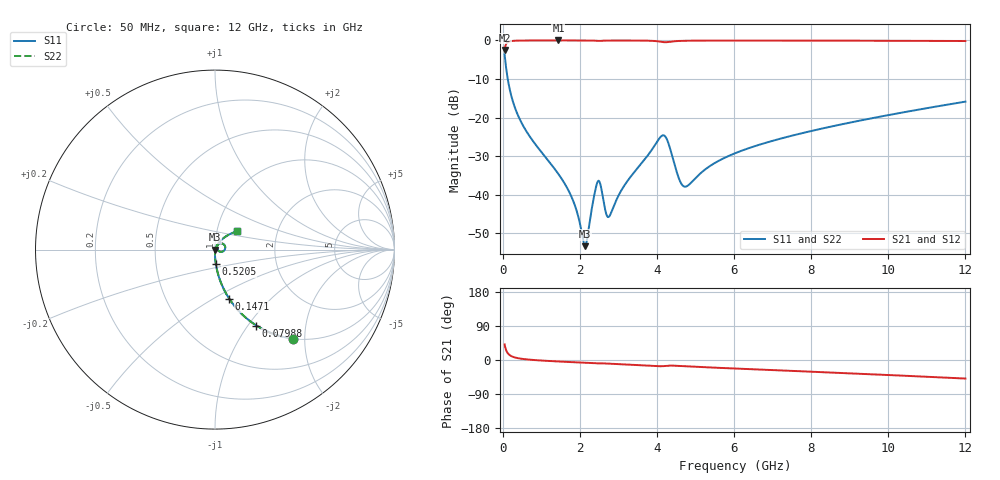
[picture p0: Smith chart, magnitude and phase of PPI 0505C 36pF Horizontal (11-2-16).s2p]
# MHz S MA R 50
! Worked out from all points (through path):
!   1601 points, 50 MHz to 12 GHz, reference 50 ohm
!   highest |S21| = -0.01 dB at 1.447 GHz (marker M1); lowest = -2.5 dB at 50 MHz (marker M2)
!   group delay of S21, straight-line fit = 12.2 ps
!   lowest |S11| = -53.3 dB at 2.134 GHz (marker M3), VSWR 1.00, Z = 50.2 - j0.0716 ohm
!   |S11| at or under -10 dB: 131.4 MHz to end of sweep
!   |S22| runs from -53.3 to -3.6 dB; largest |S21 - S12| = 0
!   S11 on the Smith chart (normalised r, x): 50 MHz: 1.00, -1.75; 79.88 MHz: 1.00, -1.10; 147.1 MHz: 1.00, -0.59; 520.5 MHz: 1.00, -0.16; 12 GHz: 1.25, +0.26
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50  0.6599 -48.9  0.7511 41.1  0.7511 41.1  0.6599 -48.9
79.875  0.4815 -61.5  0.8761 28.5  0.8761 28.5  0.4815 -61.5
147.0938  0.2852 -73.9  0.958 16.1  0.958 16.1  0.2852 -73.9
296.4688  0.1443 -82.5  0.9889 7.3  0.9889 7.3  0.1443 -82.5
520.5312  0.08008 -86.7  0.996 2.8  0.996 2.8  0.08008 -86.7
1446.656  0.01856 -90.1  0.9985 -3.9  0.9985 -3.9  0.01856 -90.1
1820.094  0.008563 -85.9  0.9984 -5.8  0.9984 -5.8  0.008563 -85.9
2044.156  0.003369 -64.3  0.9981 -6.9  0.9981 -6.9  0.003369 -64.3
2133.781  0.002163 -19.3  0.9977 -7.3  0.9977 -7.3  0.002163 -19.3
2462.406  0.01476 20.3  0.9869 -8.9  0.9869 -8.9  0.01476 20.3
2529.625  0.01392 -5.1  0.9859 -8.8  0.9859 -8.8  0.01392 -5.1
2679  0.005807 -3.2  0.9941 -9.3  0.9941 -9.3  0.005807 -3.2
2761.156  0.005239 26.1  0.9956 -9.7  0.9956 -9.7  0.005239 26.1
3157  0.01325 65.0  0.9966 -11.6  0.9966 -11.6  0.01325 65.0
4038.312  0.05167 41.8  0.9715 -16.4  0.9715 -16.4  0.05167 41.8
4239.969  0.05469 0.5  0.947 -15.4  0.947 -15.4  0.05469 0.5
4576.062  0.016 -11.3  0.9838 -15.7  0.9838 -15.7  0.016 -11.3
4725.438  0.01274 16.3  0.989 -16.6  0.989 -16.6  0.01274 16.3
6025  0.03453 60.9  0.9951 -22.5  0.9951 -22.5  0.03453 60.9
8019.156  0.06738 55.9  0.9935 -31.0  0.9935 -31.0  0.06738 55.9
10013.31  0.1081 48.2  0.9895 -39.7  0.9895 -39.7  0.1081 48.2
12000  0.161 39.4  0.9816 -48.9  0.9816 -48.9  0.161 39.4
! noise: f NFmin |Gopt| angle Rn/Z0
50  0.0003971  0.8674  0.6845  0.000644
1372  0.004093  0.6814  4.821  0.002482
2701  0.01189  0.7729  9.294  0.01062
4031  0.03258  0.8702  13.8  0.05329
5360  0.01642  0.6924  18.22  0.01015
6682  0.01586  0.6227  22.41  0.007573
8012  0.01734  0.597  26.54  0.007521
9341  0.01924  0.5848  30.56  0.007908
1.067e+04  0.02134  0.5795  34.46  0.008478
1.2e+04  0.02361  0.5789  38.23  0.009176
